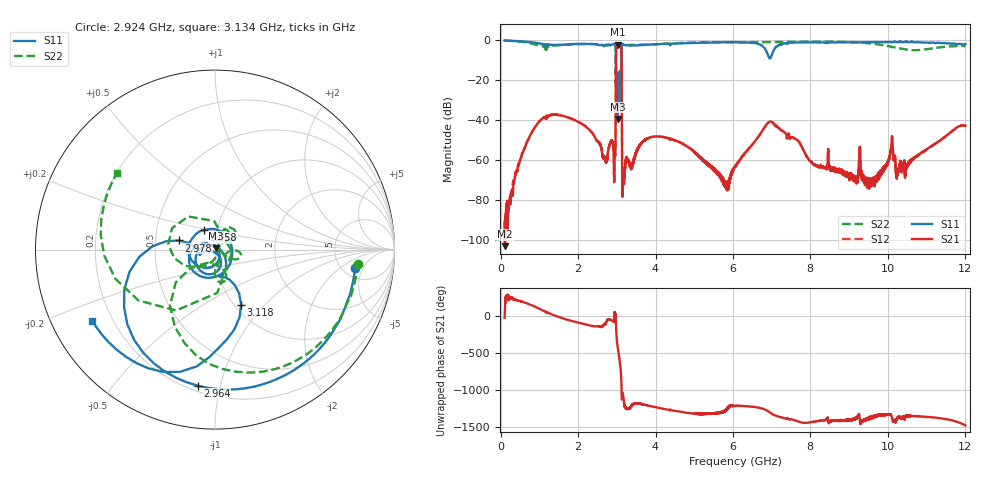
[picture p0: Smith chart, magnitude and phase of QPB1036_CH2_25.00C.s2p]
! TDS: K:\Engsetup\Winsaw\QPB1036_ALL
! Channel 1
! Ports=1 2
! seg 1=100.000000 1100.000000 101
! seg 2=1101.000000 1501.000000 401
! seg 3=1502.000000 2502.000000 101
! seg 4=2503.000000 3803.000000 1301
! seg 5=3804.000000 5004.000000 121
! seg 6=5005.000000 6005.000000 1001
! seg 7=6006.000000 8406.000000 241
! seg 8=8407.000000 10607.000000 2201
! seg 9=10608.000000 12008.000000 141
! Points=5609
! FailCode=0
! Topology=ALL_SE(12)
!VNA Cal loaded =QPB1036_ALL_25C
!PS1(V)= 5.000
!PS(mA)= 0.500
!PS2(V)= 0.630
!PS(mA)= -0.100
!PS3(V)= 1.170
!PS(mA)= 0.100
!PS4(V)= 0.630
!PS(mA)= -0.100
!Temp (C)= 25.00
# MHz S DB R 50
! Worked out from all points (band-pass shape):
!   5609 points, 100 MHz to 12.01 GHz, reference 50 ohm
!   highest |S21| = -2.37 dB at 3.032 GHz (marker M1); lowest = -103.3 dB at 110 MHz (marker M2)
!   |S21| within 3 dB of the highest: 2.985 GHz to 3.117 GHz (132.8 MHz wide, 4.35 % of centre)
!   lowest |S11| = -39.6 dB at 3.021 GHz (marker M3), VSWR 1.02, Z = 50.7 + j0.767 ohm
!   |S11| at or under -10 dB: 2.976 GHz to 3.118 GHz (141.2 MHz wide, 4.64 % of centre)
!   |S22| runs from -32.8 to -0.3 dB; largest |S21 - S12| = 0.0068
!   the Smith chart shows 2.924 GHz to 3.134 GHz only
!   S11 on the Smith chart (normalised r, x): 2.924 GHz: 6.44, -3.50; 2.964 GHz: 0.23, -0.85; 2.978 GHz: 0.66, +0.07; 3.058 GHz: 0.86, +0.19; 3.118 GHz: 1.07, -0.75; 3.134 GHz: 0.13, -0.27
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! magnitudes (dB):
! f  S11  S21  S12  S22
! 100 MHz  -0.3  -91.5  -90.4  -0.3
! 110 MHz  -0.3  -103.3  -103.2  -0.3
! 1.123 GHz  -2.2  -39.0  -39.0  -3.4
! 2.092 GHz  -2.0  -42.0  -42.0  -2.1
! 2.924 GHz  -2.1  -61.4  -61.5  -1.9
! 2.964 GHz  -2.3  -54.7  -54.6  -3.0
! 2.978 GHz  -13.7  -10.1  -10.1  -14.5
! 3.021 GHz  -39.6  -2.5  -2.5  -21.2
! 3.032 GHz  -20.7  -2.4  -2.4  -31.1
! 3.058 GHz  -18.0  -2.6  -2.6  -16.3
! 3.098 GHz  -22.0  -3.1  -3.1  -19.1
! 3.118 GHz  -9.4  -5.7  -5.7  -12.7
! 3.134 GHz  -2.0  -58.8  -58.9  -3.2
! 3.165 GHz  -2.3  -66.1  -67.3  -2.7
! 4.074 GHz  -2.1  -48.4  -48.5  -2.2
! 5.833 GHz  -1.2  -74.3  -72.6  -1.2
! 6.056 GHz  -1.1  -63.4  -63.5  -1.2
! 7.016 GHz  -6.9  -41.3  -41.2  -1.1
! 8.046 GHz  -1.2  -61.8  -61.4  -0.9
! 9.577 GHz  -1.2  -70.8  -72.8  -1.8
! 10.02 GHz  -1.0  -60.4  -60.2  -3.2
! 12.01 GHz  -2.2  -43.0  -43.0  -3.1
